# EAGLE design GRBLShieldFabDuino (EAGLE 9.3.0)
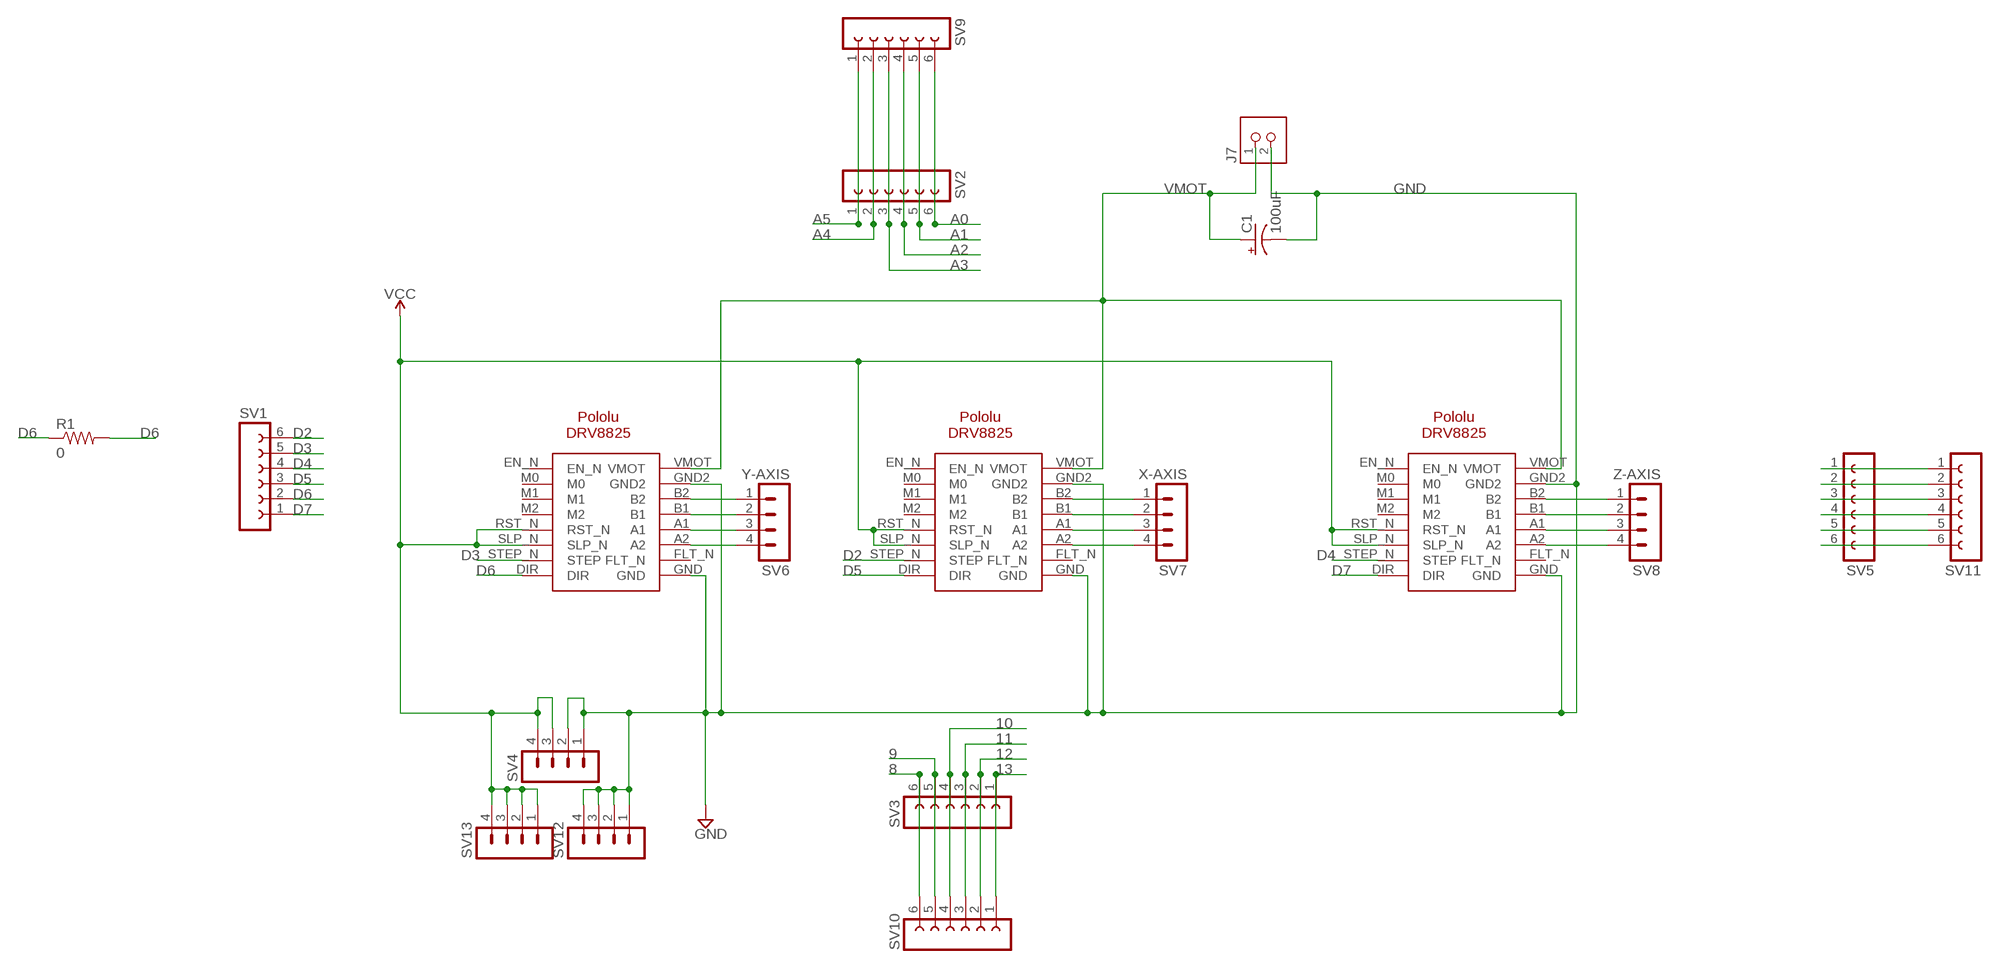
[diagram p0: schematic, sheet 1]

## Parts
C1  100uF  100UF-POLAR-RADIAL-2.5MM-25V-20%  [CPOL-RADIAL-2.5MM-6.5MM]
J7  TERM-1X02-FABLAB  [ED555DS-2DS]
R1  0  RES-US1206FAB  [R1206FAB]
SV1  FE06-1  [FE06]
SV2  FE06-1  [FE06]
SV3  FE06-1  [FE06]
SV4  MA04-1  [MA04-1]
SV5  FE06-1  [FE06]
SV6  Y-AXIS  MA04-1  [MA04-1]
SV7  X-AXIS  MA04-1  [MA04-1]
SV8  Z-AXIS  MA04-1  [MA04-1]
SV9  FE06-1  [FE06]
SV10  FE06-1  [FE06]
SV11  FE06-1  [FE06]
SV12  MA04-1  [MA04-1]
SV13  MA04-1  [MA04-1]
X-AXIS  POLOLU-DRV8825  [POLOLU-DRV8825]
Y-AXIS  POLOLU-DRV8825  [POLOLU-DRV8825]
Z-AXIS  POLOLU-DRV8825  [POLOLU-DRV8825]

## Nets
8: SV3.6 SV10.6
9: SV3.5 SV10.5
10: SV3.4 SV10.4
11: SV3.3 SV10.3
12: SV3.2 SV10.2
13: SV3.1 SV10.1
A0: SV2.6 SV9.6
A1: SV2.5 SV9.5
A2: SV2.4 SV9.4
A3: SV2.3 SV9.3
A4: SV2.2 SV9.2
A5: SV2.1 SV9.1
D2: SV1.6 X-AXIS.STEP_N(STEP)
D3: SV1.5 Y-AXIS.STEP_N(STEP)
D4: SV1.4 Z-AXIS.STEP_N(STEP)
D5: SV1.3 X-AXIS.DIR
D6: R1.1 R1.2 SV1.2 Y-AXIS.DIR
D7: SV1.1 Z-AXIS.DIR
GND: C1.2(-) J7.2 SV4.1 SV4.2 SV12.1 SV12.2 SV12.3 SV12.4 X-AXIS.GND X-AXIS.GND2 Y-AXIS.GND Y-AXIS.GND2 Z-AXIS.GND Z-AXIS.GND2
N$1: SV8.1 Z-AXIS.B2
N$2: SV8.2 Z-AXIS.B1
N$3: SV8.3 Z-AXIS.A1
N$4: SV8.4 Z-AXIS.A2
N$5: SV7.1 X-AXIS.B2
N$6: SV7.2 X-AXIS.B1
N$7: SV7.3 X-AXIS.A1
N$8: SV7.4 X-AXIS.A2
N$9: SV6.1 Y-AXIS.B2
N$10: SV6.2 Y-AXIS.B1
N$11: SV6.3 Y-AXIS.A1
N$12: SV6.4 Y-AXIS.A2
N$13: SV5.1 SV11.1
N$14: SV5.2 SV11.2
N$15: SV5.3 SV11.3
N$16: SV5.4 SV11.4
N$17: SV5.5 SV11.5
N$18: SV5.6 SV11.6
VCC: SV4.3 SV4.4 SV13.1 SV13.2 SV13.3 SV13.4 X-AXIS.RST_N X-AXIS.SLP_N Y-AXIS.RST_N Y-AXIS.SLP_N Z-AXIS.RST_N Z-AXIS.SLP_N
VMOT: C1.1(+) J7.1 X-AXIS.VMOT Y-AXIS.VMOT Z-AXIS.VMOT
Unconnected: X-AXIS.EN_N X-AXIS.FLT_N X-AXIS.M0 X-AXIS.M1 X-AXIS.M2 Y-AXIS.EN_N Y-AXIS.FLT_N Y-AXIS.M0 Y-AXIS.M1 Y-AXIS.M2 Z-AXIS.EN_N Z-AXIS.FLT_N Z-AXIS.M0 Z-AXIS.M1 Z-AXIS.M2

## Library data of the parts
C1 = SparkFun-Capacitors:100UF-POLAR: 100µF polarized capacitors; PROD_ID: CAP-08439
J7 = fab:TERM-1X02: 3.5mm terminal block, 2 positions ED555-2DS as found in the fablab inventory.
R1 = fab:RES-US: Resistor (US Symbol)
SV1-SV3 SV5 SV9-SV11 = con-lsta:FE06-1: FEMALE HEADER; OC_FARNELL: unknown; OC_NEWARK: unknown
SV4 SV6-SV8 SV12 SV13 = con-lstb:MA04-1: PIN HEADER; OC_FARNELL: unknown; OC_NEWARK: unknown
X-AXIS Y-AXIS Z-AXIS = alvarop-lib:POLOLU-DRV8825

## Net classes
0 default: clearance 0.406 mm

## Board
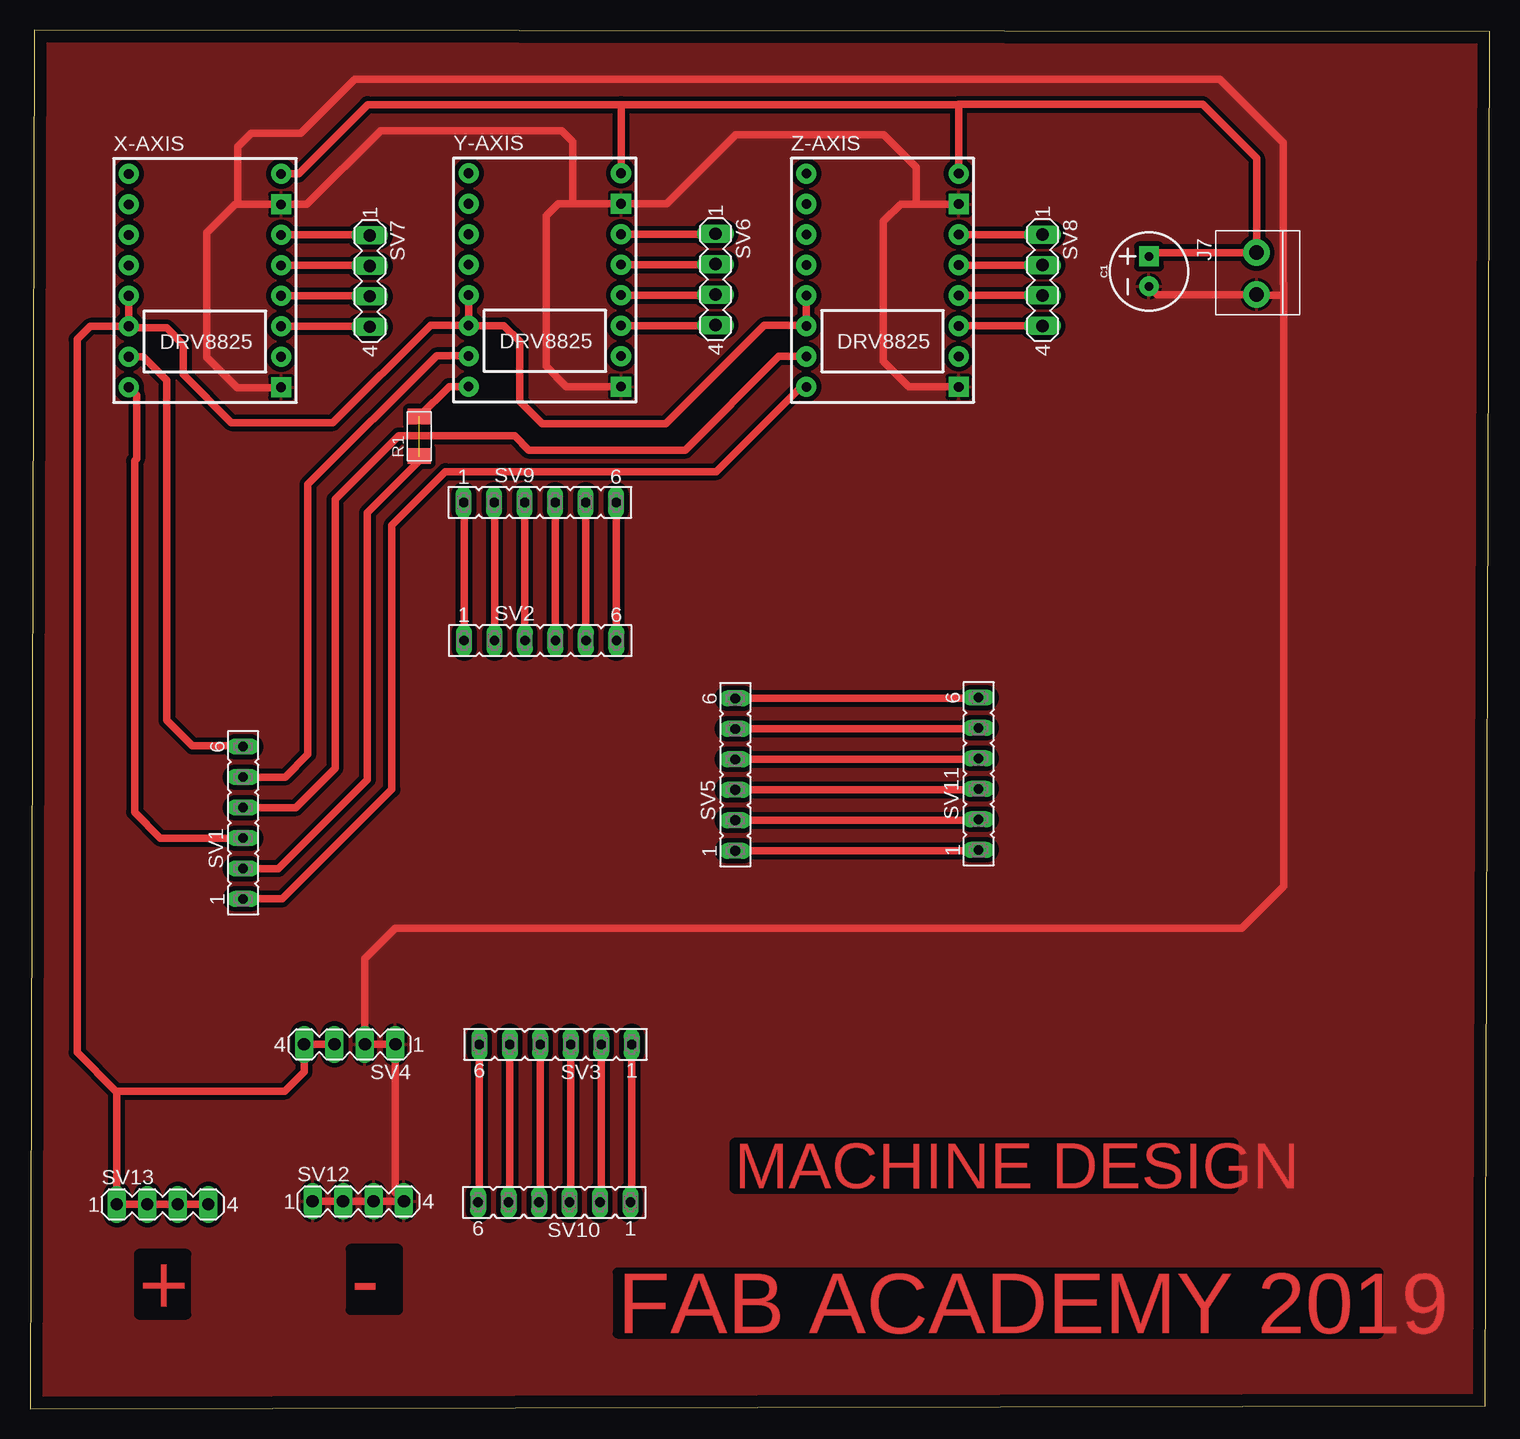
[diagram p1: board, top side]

Size 121.65 x 114.91 mm. Coordinates in mm from the lower left corner, seen from the top.
Outline: 0,0 121.29,0.28 121.65,114.78 0.36,114.91 0,0
Copper layers (1*16): Top 0.035mm / dielectric 1.5mm / Bottom 0.035mm
Design rules "default": minimum track width 6mil, minimum drill 0.35mm, track to track 6mil, track to pad 6mil, pad to pad 6mil, via to via 6mil, smd to smd 6mil, copper to edge 40mil, drill to drill 6mil, minimum pad ring 10mil, minimum via ring 8mil, stop-mask expansion 4mil, vias tented up to drill 0mil, thermal gap 10mil

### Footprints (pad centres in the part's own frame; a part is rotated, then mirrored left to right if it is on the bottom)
CPOL-RADIAL-2.5MM-6.5MM = drill 0.7 pad 1.651 square: 1 1.25,0 | drill 0.7 pad 1.651: 2 -1.25,0
ED555DS-2DS = drill 1.2 pad 2.184: 1 1.8,0; 2 -1.7,0
R1206FAB = smd 1.27 x 1.905: 1 -1.651,0; 2 1.651,0
FE06 = drill 0.813 long: 1 -6.35,0; 2 -3.81,0; 3 -1.27,0; 4 1.27,0; 5 3.81,0; 6 6.35,0
MA04-1 = drill 1.016 long: 1 -3.81,0; 2 -1.27,0; 3 1.27,0; 4 3.81,0
POLOLU-DRV8825 = drill 0.8 pad 1.676: A1 6.35,-1.27; A2 6.35,-3.81; B1 6.35,1.27; B2 6.35,3.81; DIR -6.35,-8.89; EN_N -6.35,8.89; FLT_N 6.35,-6.35; M0 -6.35,6.35; M1 -6.35,3.81; M2 -6.35,1.27; RST_N -6.35,-1.27; SLP_N -6.35,-3.81; STEP_N -6.35,-6.35; VMOT 6.35,8.89 | drill 0.8 pad 1.676 square: GND 6.35,-8.89; GND2 6.35,6.35

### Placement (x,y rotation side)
C1  93.24,94.79 90 top
J7  102.21,94.56 90 top
R1  32.44,81.05 90 top
SV1  17.75,48.84 90 top
SV2  42.52,64.03 0 top
SV3  43.79,30.38 180 top
SV4  26.64,30.38 180 top
SV5  58.78,52.86 90 top
SV6  57.12,94.13 270 top
SV7  28.32,93.98 270 top
SV8  84.38,94.06 270 top
SV9  42.49,75.54 0 top
SV10  43.69,17.22 180 top
SV11  79.04,52.93 90 top
SV12  27.36,17.3 0 top
SV13  11.05,17.04 0 top
X-AXIS  14.58,94.03 0 top
Y-AXIS  42.9,94.08 0 top
Z-AXIS  71.04,94.06 0 top

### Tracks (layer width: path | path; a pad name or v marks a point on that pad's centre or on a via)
8
  Top 0.61: SV3.6 37.44,17.32 SV10.6
9
  Top 0.61: SV3.5 39.98,17.32 SV10.5
10
  Top 0.61: SV3.4 42.52,17.32 SV10.4
11
  Top 0.61: SV3.3 45.06,17.32 SV10.3
12
  Top 0.61: SV3.2 47.6,17.32 SV10.2
13
  Top 0.61: SV3.1 50.14,17.32 SV10.1
A0
  Top 0.61: SV2.6 48.87,75.51 SV9.6
A1
  Top 0.61: SV2.5 46.33,75.51 SV9.5
A2
  Top 0.61: SV2.4 43.79,75.51 SV9.4
A3
  Top 0.61: SV2.3 41.25,75.51 SV9.3
A4
  Top 0.61: SV2.2 38.71,75.51 SV9.2
A5
  Top 0.61: SV2.1 36.17,75.51 SV9.1
D2
  Top 0.61: X-AXIS.STEP_N 9.45,87.68 11.4,85.73 11.4,57.38 13.54,55.25 17.7,55.25 SV1.6
D3
  Top 0.61: Y-AXIS.STEP_N 36.52,87.76 33.88,87.76 23.16,77.04 23.16,54.56 21.26,52.65 SV1.5
D4
  Top 0.61: SV1.4 22.15,50.11 25.43,53.39 25.43,75.79 30.71,81.08 40.39,81.08 41.55,79.91 54.61,79.91 62.41,87.71 Z-AXIS.STEP_N
D5
  Top 0.61: X-AXIS.DIR 8.89,84.48 8.89,79.17 8.71,78.99 8.71,49.73 10.87,47.57 SV1.3
D6  (1 unrouted)
  Top 0.61: Y-AXIS.DIR 34.92,85.19 R1.2 | R1.1 32.44,78.99 28.12,74.68 28.12,52.45 20.7,45.03 SV1.2
D7
  Top 0.61: SV1.1 21.01,42.49 30.15,51.64 30.15,73.63 34.62,78.11 57.2,78.11 64.26,85.17 Z-AXIS.DIR
GND
  Top 0.61: 45.24,100.43 Y-AXIS.GND2 53.06,100.43 58.83,106.2 71.15,106.2 73.86,103.48 73.86,100.41 | 45.24,100.43 44.02,100.43 43,99.42 43,86.89 44.7,85.19 Y-AXIS.GND | Z-AXIS.GND2 73.86,100.41 | 73.86,100.41 72.54,100.41 71.09,98.96 71.09,87.3 73.23,85.17 Z-AXIS.GND | 17.3,100.38 X-AXIS.GND2 23.06,100.38 29.21,106.53 44.32,106.53 45.24,105.61 45.24,100.43 | 17.3,100.38 17.09,100.38 14.73,98.02 14.73,87.66 17.27,85.12 20.9,85.12 X-AXIS.GND | 17.3,100.38 17.3,105.18 18.44,106.32 22.58,106.32 27.08,110.82 99.14,110.82 104.44,105.51 104.44,93.79 104.47,93.76 104.47,92.81 | 104.47,92.81 104.47,43.56 100.96,40.06 30.45,40.06 27.91,37.52 SV4.2 SV4.1 30.45,18.01 SV12.4 SV12.3 SV12.2 SV12.1 | 104.47,92.81 104.44,92.84 | 104.47,92.81 102.26,92.81 J7.2 93.92,92.86 C1.2
  pour Top: -0.1,114.35 120.09,114.35 121.23,113.21 121.23,0.43 120.9,0.1 -0.1,0.1
N$1
  Top 0.61: Z-AXIS.B2 SV8.1
N$2
  Top 0.61: Z-AXIS.B1 SV8.2
N$3
  Top 0.61: Z-AXIS.A1 SV8.3
N$4
  Top 0.61: Z-AXIS.A2 SV8.4
N$5
  Top 0.61: X-AXIS.B2 28.27,97.84 SV7.1
N$6
  Top 0.61: X-AXIS.B1 28.27,95.3 SV7.2
N$7
  Top 0.61: X-AXIS.A1 28.27,92.76 SV7.3
N$8
  Top 0.61: X-AXIS.A2 28.27,90.22 SV7.4
N$9
  Top 0.61: Y-AXIS.B2 57.07,97.89 SV6.1
N$10
  Top 0.61: Y-AXIS.B1 57.07,95.35 SV6.2
N$11
  Top 0.61: Y-AXIS.A1 57.07,92.81 SV6.3
N$12
  Top 0.61: Y-AXIS.A2 57.07,90.27 SV6.4
N$13
  Top 0.61: SV5.1 78.97,46.51 SV11.1
N$14
  Top 0.61: SV5.2 78.97,49.05 SV11.2
N$15
  Top 0.61: SV5.3 78.97,51.59 SV11.3
N$16
  Top 0.61: SV5.4 78.97,54.13 SV11.4
N$17
  Top 0.61: SV5.5 78.97,56.67 SV11.5
N$18
  Top 0.61: SV5.6 78.97,59.21 SV11.6
VCC
  Top 0.61: SV4.3 SV4.4 22.83,28.09 21.23,26.49 7.16,26.49 | X-AXIS.SLP_N X-AXIS.RST_N | Y-AXIS.SLP_N Y-AXIS.RST_N | Z-AXIS.RST_N Z-AXIS.SLP_N 64.64,90.3 61.19,90.3 52.98,82.09 42.67,82.09 40.79,83.97 40.79,88.98 39.5,90.27 36.96,90.27 | 36.58,90.3 Y-AXIS.SLP_N | Y-AXIS.SLP_N 36.96,90.27 | X-AXIS.SLP_N 8.36,90.09 11.38,90.09 12.78,88.7 12.78,86.21 16.79,82.19 25.25,82.19 33.38,90.32 36.91,90.32 36.96,90.27 | X-AXIS.SLP_N 5.03,90.22 3.94,89.13 3.94,29.72 7.16,26.49 | SV13.4 SV13.3 SV13.2 SV13.1 7.24,26.42 7.16,26.49
VMOT
  Top 0.61: X-AXIS.VMOT 22.38,102.92 28.14,108.69 49.25,108.69 | Y-AXIS.VMOT 49.25,108.69 | Z-AXIS.VMOT 77.39,108.69 | 77.39,108.69 77.39,108.71 97.71,108.71 102.21,104.22 J7.1 93.56,96.36 C1.1 | 49.25,108.69 77.39,108.69

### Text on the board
Top: MACHINE DESIGN | - | + | FAB ACADEMY 2019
